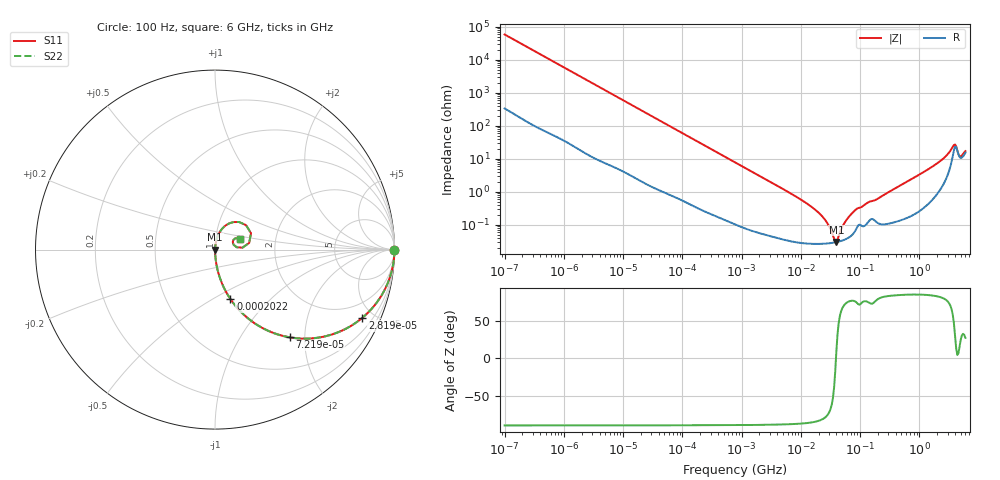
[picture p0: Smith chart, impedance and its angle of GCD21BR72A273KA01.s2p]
!Murata Part Number: GCD21BR72A273KA01
!These Parameters are Measured in Series Mode Connection
!Data Generated on Mar 13, 2026
!  o--ll--o
!Port1  Port2
!  o------o
!Operation Temp=25[degC], DC Bias Voltage=0[V]
!Freq. Start=100[Hz] Stop=6[GHz] 401[Steps]
# Hz S RI R 50
!Freq.(Hz) S11(Real) S11(Imag) S21(Real) S21(Imag) S12(Real) S12(Imag) S22(Real) S22(Imag)
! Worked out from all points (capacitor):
!   401 points, 100 Hz to 6 GHz, reference 50 ohm
!   read as one part in series: C = 26.8 nF near 109 Hz
!   lowest |Z| = 30.5 mohm at 39.84 MHz (marker M1)
!   series resonance near 39.23 MHz, so ESL is about 610 pH
!   S11 on the Smith chart (normalised r, x): 100 Hz: open; 28.19 kHz: 1.03, -4.30; 72.19 kHz: 1.01, -1.69; 202.2 kHz: 1.01, -0.61; 6 GHz: 1.31, +0.16
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100  1 -0.00169  1.25e-05 0.00169  1.25e-05 0.00169  1 -0.00169
2008  0.9987 -0.0335  0.00131 0.0335  0.00131 0.0335  0.9987 -0.0335
8416  0.98 -0.1367  0.02 0.1367  0.02 0.1367  0.98 -0.1367
28191  0.8202 -0.3805  0.1798 0.3805  0.1798 0.3805  0.8202 -0.3805
40335  0.6921 -0.4579  0.3079 0.4579  0.3079 0.4579  0.6921 -0.4579
72189  0.416 -0.4886  0.584 0.4886  0.584 0.4886  0.416 -0.4886
202169  0.0861 -0.2758  0.9139 0.2758  0.9139 0.2758  0.0861 -0.2758
774597  0.00732 -0.079  0.9927 0.079  0.9927 0.079  0.00732 -0.079
1.555665e7  0.000279 -0.00341  0.9997 0.00341  0.9997 0.00341  0.000279 -0.00341
2.545746e7  0.000273 -0.00143  0.9997 0.00143  0.9997 0.00143  0.000273 -0.00143
3.045065e7  0.000279 -0.000823  0.9997 0.000823  0.9997 0.000823  0.000279 -0.000823
3.64232e7  0.000292 -0.000238  0.9997 0.000238  0.9997 0.000238  0.000292 -0.000238
3.983537e7  0.000301 5.04e-05  0.9997 -5.04e-05  0.9997 -5.04e-05  0.000301 5.04e-05
5.699437e7  0.00037 0.00125  0.9996 -0.00125  0.9996 -0.00125  0.00037 0.00125
8.154455e7  0.000637 0.00266  0.9994 -0.00266  0.9994 -0.00266  0.000637 0.00266
3.124326e8  0.0012 0.0101  0.9988 -0.0101  0.9988 -0.0101  0.0012 0.0101
1.873145e9  0.0118 0.066  0.9882 -0.066  0.9882 -0.066  0.0118 0.066
2.931063e9  0.0429 0.1196  0.9571 -0.1196  0.9571 -0.1196  0.0429 0.1196
3.666503e9  0.1342 0.1536  0.8658 -0.1536  0.8658 -0.1536  0.1342 0.1536
4.009986e9  0.2006 0.0915  0.7994 -0.0915  0.7994 -0.0915  0.2006 0.0915
5.016141e9  0.0989 0.0418  0.9011 -0.0418  0.9011 -0.0418  0.0989 0.0418
6e9  0.1371 0.0602  0.8629 -0.0602  0.8629 -0.0602  0.1371 0.0602
